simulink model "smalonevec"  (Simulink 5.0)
settings: Solver=ode23t  StartTime=0.0  StopTime=10  MaxStep=0.02  RelTol=1e-5  AbsTol=1e-4
InitFcn:
  | smalonevecdef
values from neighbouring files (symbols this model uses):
  Ef = parEf(m)    [Ccurverun.m]
  Ra = .95    (= 0.95)    [altwdgs.m]    (also in Ccurverun.m = 0.018)
  wo = 2*pi*freq0    [calc0.m]    (also in IMabc2.m = 376.991118431; imabcparam.m = 376.991118431; IMabcrun0.m = 376.991118431; IMabcrun1.m = 376.991118431)
undefined symbols (not defined in the file or in its folder): fa0, fk0, L_1, phif0, Rf, Rkd, Rkq, vf0

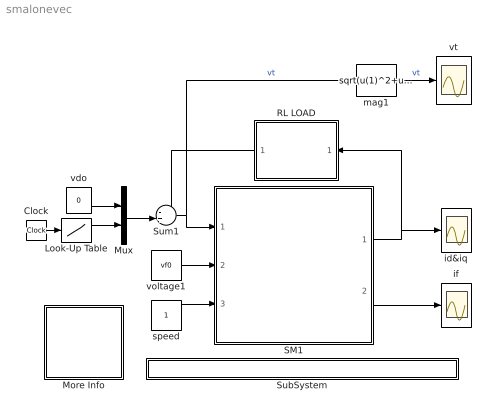
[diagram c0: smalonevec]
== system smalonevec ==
  Clock : Clock
  Look-Up Table : Lookup  InputValues=[0 0.5 0.51 20]  OutputValues=[Ef Ef 0 0]
  More Info : Subsystem
  Mux : Mux  Inputs=2
  RL LOAD : Subsystem  Orientation=left  mask{Rline=0.4, Lline=1, wo=2*pi*60}
      mask prompts: Rline "Rline [ pu]"; Lline "Lline [pu]"; wo "wo [rad/s]"
  SM1 : Subsystem
  SubSystem : Subsystem
  Sum1 : Sum  Inputs=-+|
  id&iq : Scope
  if : Scope
  mag1 : Fcn  Expr=sqrt(u(1)^2+u(2)^2)
  speed : Constant
  vdo : Constant  Value=0
  voltage1 : Constant  Value=vf0
  vt : Scope
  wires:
  voltage1/1 -> SM1/2(vf)
  SM1/2(if) -> if/1
  speed/1 -> SM1/3(wm)
  Look-Up Table/1 -> Mux/2
  Mux/1 -> Sum1/2
  RL LOAD/1(v_out) -> Sum1/1
  Sum1/1 -> SM1/1(vs), mag1/1  "vt"
  SM1/1(ia) -> RL LOAD/1(i_in), id&iq/1
  mag1/1 -> vt/1  "vt"
  vdo/1 -> Mux/1
  Clock/1 -> Look-Up Table/1

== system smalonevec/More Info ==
  note: The generator runs under open-cicuit conditions when an inductive-resistive load is suddenly applied
  note: Synchronous generator voltage dip

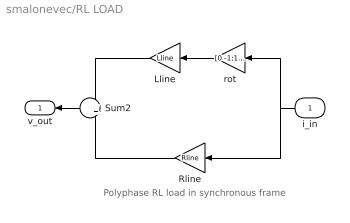
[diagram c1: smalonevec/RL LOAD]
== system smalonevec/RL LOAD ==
  note: Polyphase RL load in synchronous frame
  i_in : Inport  Orientation=left
  Lline : Gain  Orientation=left  Gain=Lline
  Rline : Gain  Orientation=left  Gain=Rline
  Sum2 : Sum  Orientation=left
  rot : Gain  Orientation=left  Gain=[0 -1;1 0]  Multiplication=Matrix(K*u)
  v_out : Outport  Orientation=left
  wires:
  Sum2/1 -> v_out/1
  i_in/1 -> rot/1, Rline/1
  rot/1 -> Lline/1
  Lline/1 -> Sum2/1
  Rline/1 -> Sum2/2

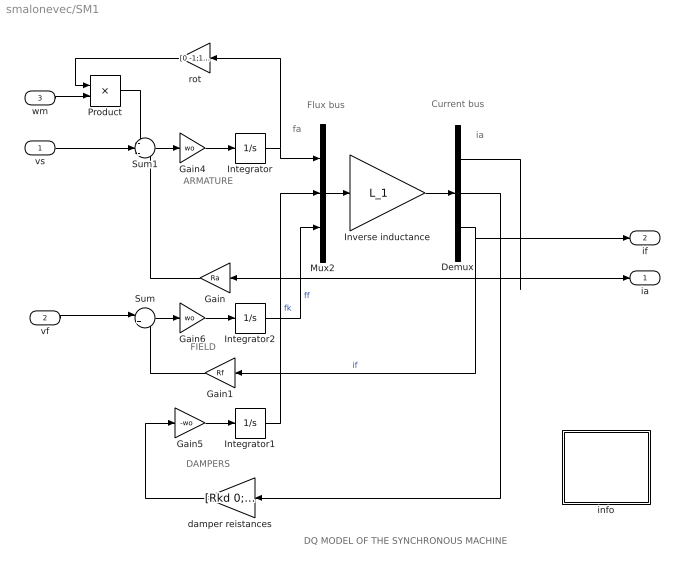
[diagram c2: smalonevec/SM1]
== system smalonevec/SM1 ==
  note: DAMPERS
  note: ARMATURE
  note: fa
  note: ia
  note: FIELD
  note: DQ MODEL OF THE SYNCHRONOUS MACHINE
  note: Flux bus
  note: Current bus
  vs : Inport
  vf : Inport  Port=2
  wm : Inport  Port=3
  Demux : Demux  Outputs=3
  Gain : Gain  Orientation=left  Gain=Ra
  Gain1 : Gain  Orientation=left  Gain=Rf
  Gain4 : Gain  Gain=wo
  Gain5 : Gain  Gain=-wo
  Gain6 : Gain  Gain=wo
  Integrator : Integrator  InitialCondition=fa0
  Integrator1 : Integrator  InitialCondition=fk0
  Integrator2 : Integrator  InitialCondition=phif0
  Inverse inductance : Gain  Gain=L_1  Multiplication=Matrix(K*u)
  Mux2 : Mux  Inputs=3
  Product : Product
  Sum : Sum  Inputs=|+-
  Sum1 : Sum  Inputs=-+-
  damper reistances : Gain  Orientation=left  Gain=[Rkd 0;0 Rkq]  Multiplication=Matrix(K*u)
  info : Subsystem
  rot : Gain  Orientation=left  Gain=[0 -1;1 0]  Multiplication=Matrix(K*u)
  ia : Outport
  if : Outport  Port=2
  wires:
  Product/1 -> Sum1/1
  rot/1 -> Product/1
  wm/1 -> Product/2
  Gain5/1 -> Integrator1/1
  damper reistances/1 -> Gain5/1
  Integrator/1 -> Mux2/1, rot/1
  Sum1/1 -> Gain4/1
  Gain4/1 -> Integrator/1
  vs/1 -> Sum1/2
  Gain/1 -> Sum1/3
  Gain6/1 -> Integrator2/1
  Sum/1 -> Gain6/1
  vf/1 -> Sum/1
  Gain1/1 -> Sum/2
  Demux/1 -> Gain/1, ia/1
  Mux2/1 -> Inverse inductance/1
  Inverse inductance/1 -> Demux/1
  Integrator1/1 -> Mux2/2  "fk"
  Integrator2/1 -> Mux2/3  "ff"
  Demux/2 -> damper reistances/1
  Demux/3 -> if/1, Gain1/1  "if"

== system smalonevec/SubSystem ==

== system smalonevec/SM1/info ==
  note: This demonstration illustrates the dynamics of a synchronous generator, initially at no load, following a three-phase short circuit at the terminals.
  note: Synchronous machine transients under shortcircuit
